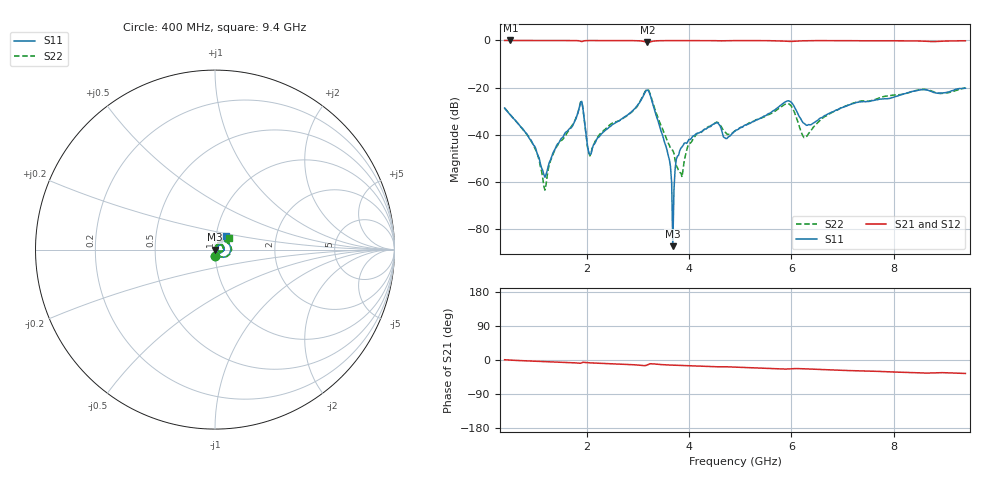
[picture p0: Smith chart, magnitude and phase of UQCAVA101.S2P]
!  Part Number  UQCAVA101	Mounting Orientation: Horizontal
!  Description: RF capacitors
!  Application: Coupling, Bypass, Tuning, DC Block
!  Filters, Matching
# GHZ S DB R 50
! Freq  |S11|  S11 Ph  |S21|  S21 Ph  |S12|  S12 Ph  |S22|  S22 Ph
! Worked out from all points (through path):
!   401 points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, 400 MHz to 9.4 GHz, reference 50 ohm
!   highest |S21| = -0.01 dB at 513 MHz (marker M1); lowest = -0.9 dB at 3.19 GHz (marker M2)
!   group delay of S21, straight-line fit = 10.9 ps
!   lowest |S11| = -87.3 dB at 3.685 GHz (marker M3), VSWR 1.00, Z = 50 - j0.00431 ohm
!   |S11| at or under -10 dB: start of sweep to end of sweep
!   |S22| runs from -63.5 to -20.1 dB; largest |S21 - S12| = 0.0067
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0.4  -28.70 -88.3  -0.02 0.7  -0.01 0.7  -28.70 -88.5
0.513  -31.60 -88.2  -0.01 -0.3  -0.01 -0.3  -31.60 -88.4
0.963  -44.32 -81.9  -0.02 -3.1  -0.01 -3.1  -44.46 -85.7
1.188  -58.06 -6.5  -0.02 -4.2  -0.01 -4.3  -63.54 -0.5
1.39  -45.89 68.3  -0.02 -5.2  -0.01 -5.3  -46.06 76.7
1.908  -25.86 -3.3  -0.47 -7.1  -0.45 -7.2  -25.87 2.1
2.065  -48.48 9.7  -0.05 -7.5  -0.03 -7.6  -49.02 20.9
3.19  -21.01 -0.2  -0.85 -12.8  -0.83 -12.9  -20.67 -0.3
3.415  -35.49 -77.5  -0.12 -11.7  -0.10 -11.8  -33.96 -65.2
3.595  -48.74 -77.3  -0.07 -13.1  -0.06 -13.2  -43.54 -56.0
3.685  -87.30 -91.8  -0.07 -13.6  -0.05 -13.7  -46.63 -37.7
3.843  -45.69 77.8  -0.06 -14.4  -0.05 -14.6  -56.27 25.9
3.955  -43.68 71.6  -0.06 -15.0  -0.04 -15.1  -46.70 102.9
4.495  -35.39 44.0  -0.10 -17.7  -0.09 -17.9  -35.28 62.9
4.72  -41.61 32.4  -0.13 -17.9  -0.11 -18.0  -39.14 42.8
4.9  -38.48 55.6  -0.07 -18.8  -0.06 -19.0  -38.40 67.4
5.913  -25.74 17.8  -0.36 -23.8  -0.35 -24.0  -26.87 24.6
6.25  -35.20 -5.8  -0.15 -23.3  -0.15 -23.5  -41.25 14.8
6.408  -35.38 27.1  -0.10 -24.2  -0.10 -24.5  -37.47 61.3
7.015  -28.33 49.0  -0.09 -27.4  -0.10 -27.6  -28.26 64.2
7.915  -24.64 47.1  -0.11 -31.2  -0.13 -31.4  -23.40 46.3
9.4  -20.29 50.0  -0.14 -35.5  -0.16 -35.9  -20.14 39.3
